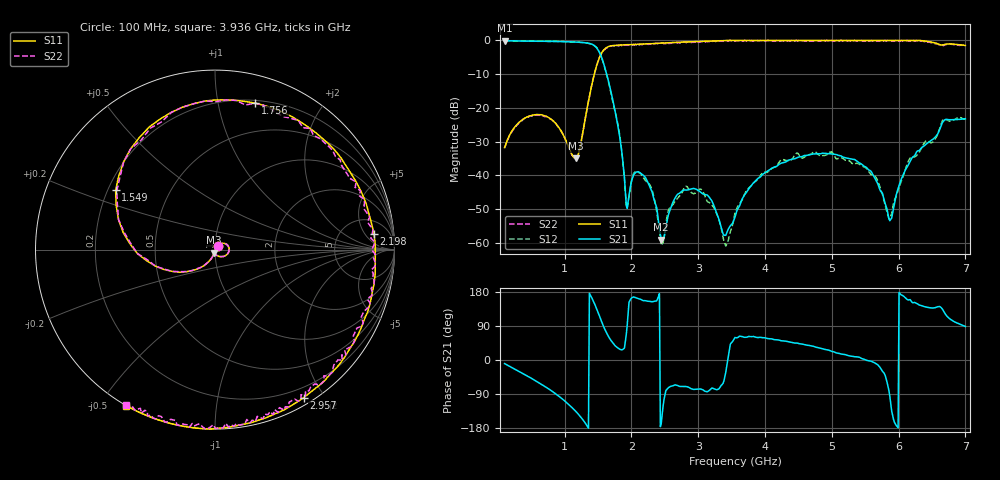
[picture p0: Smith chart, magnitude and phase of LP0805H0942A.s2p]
!	AVX	THIN	FILM	OPERATION
!	LP0805	High	Performance	Low	Pass	Filter	P/N	LP0805H0942ASTR
!	29	June	2017
#	MHZ	S	DB	R	50
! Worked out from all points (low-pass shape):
!   501 points, 100 MHz to 7 GHz, reference 50 ohm
!   highest |S21| = -0.08 dB at 100 MHz (marker M1); lowest = -59.1 dB at 2.446 GHz (marker M2)
!   |S21| within 3 dB of the highest: start of sweep to 1.507 GHz
!   lowest |S11| = -35.0 dB at 1.163 GHz (marker M3), VSWR 1.04, Z = 49.4 - j1.66 ohm
!   |S11| at or under -10 dB: start of sweep to 1.443 GHz
!   |S22| runs from -35.1 to 0.0 dB; largest |S21 - S12| = 0.023
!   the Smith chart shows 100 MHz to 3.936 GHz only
!   S11 on the Smith chart (normalised r, x): 100 MHz: 1.03, +0.04; 1.549 GHz: 0.23, +0.26; 1.756 GHz: 0.22, +1.29; 2.198 GHz: 10, +8; 2.957 GHz: 0.08, -1.76; 3.936 GHz: -0.00, -0.58
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100  -31.78 53.0  -0.08 -9.6  -0.06 -9.6  -31.88 52.8
638.2  -22.01 -4.8  -0.24 -62.5  -0.22 -62.6  -22.11 -4.8
1162.6  -34.95 -110.2  -0.48 -134.9  -0.47 -135.2  -35.15 -110.3
1259.2  -28.64 -109.2  -0.60 -154.8  -0.60 -155.2  -28.84 -109.2
1411  -12.66 -147.1  -1.14 162.2  -1.25 161.7  -12.86 -147.3
1549  -3.81 149.2  -4.81 102.8  -4.74 102.8  -3.91 149.1
1756  -1.45 74.7  -21.09 37.5  -21.25 38.5  -1.45 74.6
1935.4  -1.24 40.0  -49.78 90.9  -49.95 91.2  -1.34 40.0
2045.8  -1.17 24.0  -39.52 165.5  -39.13 162.6  -1.37 23.9
2197.6  -1.01 5.7  -40.37 156.7  -41.26 156.9  -1.11 5.6
2404.6  -0.84 -15.1  -53.86 167.7  -54.51 166.5  -0.84 -15.3
2446  -0.78 -19.0  -59.08 -166.6  -60.80 -166.7  -0.78 -19.0
2584  -0.65 -30.9  -49.89 -69.7  -49.40 -73.5  -0.85 -31.1
2956.6  -0.34 -59.1  -44.02 -77.2  -45.26 -73.8  -0.54 -59.3
3412  -0.04 -89.0  -57.79 -32.2  -61.01 -28.4  -0.04 -89.1
3550  0.00 -97.3  -52.37 59.4  -51.24 61.4  -0.20 -97.5
3936.4  0.00 -119.7  -40.35 59.8  -39.88 61.5  0.00 -119.9
4709.2  0.00 -162.7  -33.72 36.7  -33.34 34.5  -0.20 -162.8
5551  0.00 144.2  -38.39 -2.2  -38.83 2.7  -0.20 144.0
5854.6  0.00 120.6  -52.93 -80.5  -52.80 -80.5  0.00 120.4
6172  0.00 92.1  -35.87 159.4  -34.85 159.3  -0.20 92.0
7000  -1.46 7.9  -23.20 88.4  -23.39 87.5  -1.56 7.8
